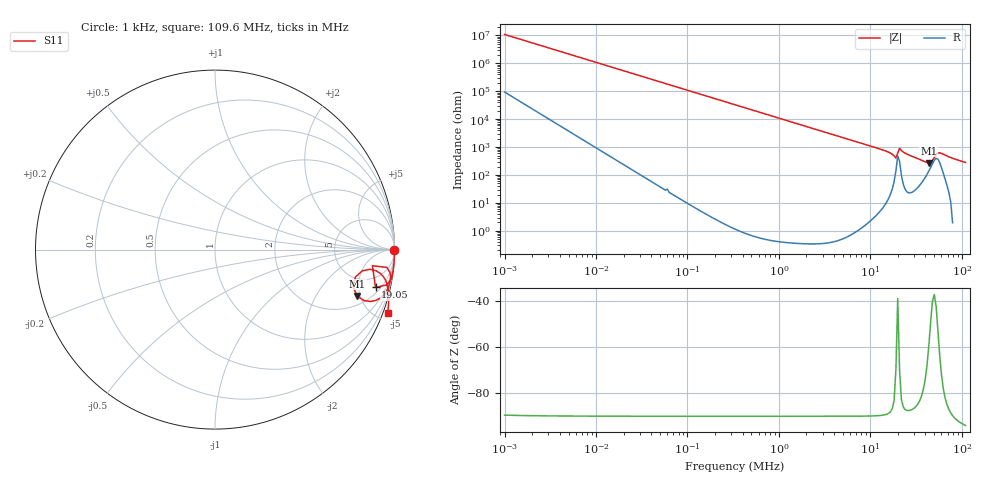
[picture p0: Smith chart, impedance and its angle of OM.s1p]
! EM Consulting and Software
! Touchstone file was created on 2026-03-05  19:00:35
# HZ S RI R 50.0000
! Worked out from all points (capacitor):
!   253 points, 1 kHz to 109.6 MHz, reference 50 ohm
!   read as one part to ground: C = 14.7 pF near 1.047 kHz
!   lowest |Z| = 273 ohm at 43.65 MHz (marker M1)
!   S11 on the Smith chart (normalised r, x): 1 kHz: open; 19.05 MHz: 2.82, -7.59; 109.6 MHz: -0.39, -5.64
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1000  1 -9.24e-06
4365.158  1 -4.03e-05
18197.01  1 -0.000168
79432.82  1 -0.000734
331131.1  1 -0.00306
1445440  0.9999 -0.0133
6025596  0.9985 -0.0551
1.148154e7  0.9942 -0.1045
1.659587e7  0.9813 -0.1621
1.819701e7  0.956 -0.1973
1.905461e7  0.8943 -0.2103
1.995262e7  0.8771 -0.0899
2.089296e7  0.9578 -0.0995
2.187762e7  0.9749 -0.128
2.630268e7  0.9741 -0.1867
3.162278e7  0.9542 -0.2337
3.630781e7  0.9177 -0.2718
3.981072e7  0.8671 -0.289
4.168694e7  0.8303 -0.284
4.365158e7  0.792 -0.2584
4.570882e7  0.77 -0.209
4.786301e7  0.7819 -0.1534
5.011872e7  0.8208 -0.1183
5.248075e7  0.8639 -0.1099
5.754399e7  0.9225 -0.134
6.606934e7  0.9567 -0.1863
8.317638e7  0.9683 -0.2614
1.096478e8  0.9622 -0.3507
